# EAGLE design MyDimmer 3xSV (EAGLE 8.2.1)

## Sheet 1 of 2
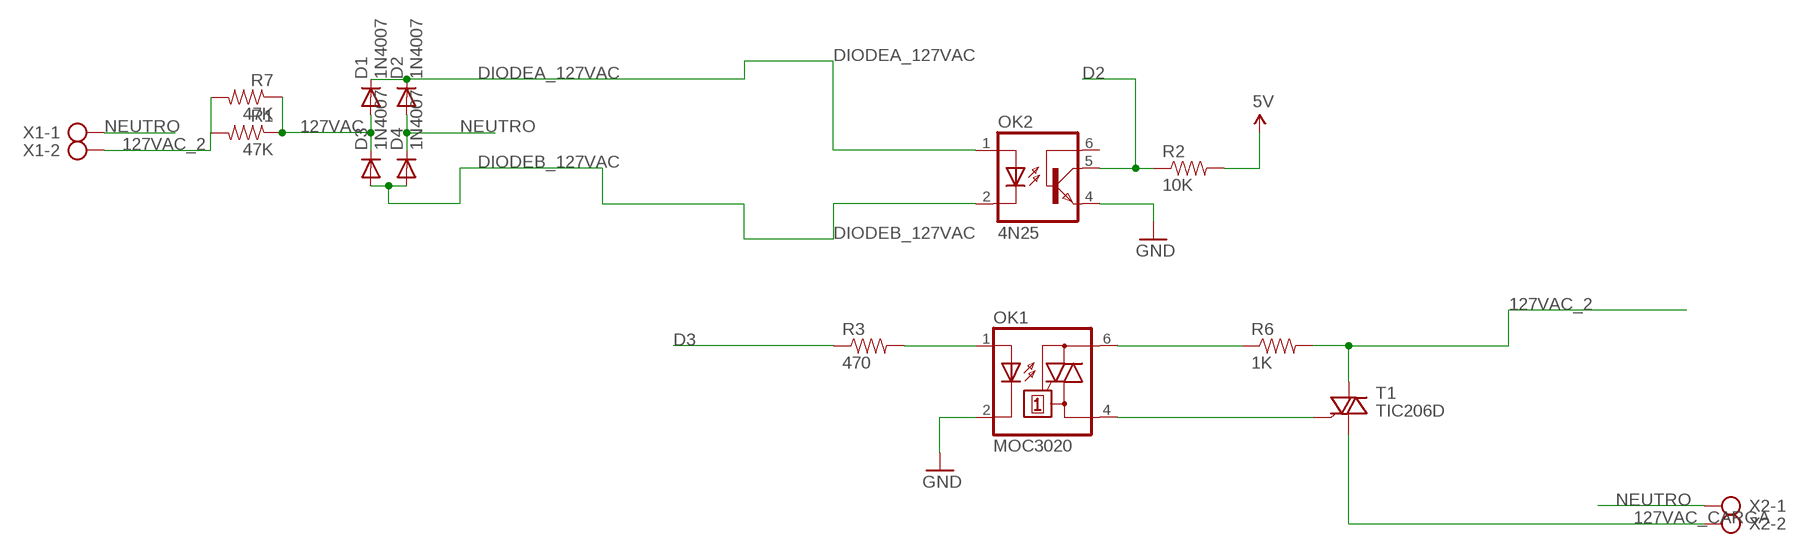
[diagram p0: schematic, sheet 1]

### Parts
D1  1N4007  1N4004  [DO41-10]
D2  1N4007  1N4004  [DO41-10]
D3  1N4007  1N4004  [DO41-10]
D4  1N4007  1N4004  [DO41-10]
OK1  MOC3020  MOC3021M  [DIL06]
OK2  4N25  4N25M  [DIL06]
R1  47K  RESISTORPTH-1/4W  [AXIAL-0.4]
R2  10K  RESISTORPTH-1/4W  [AXIAL-0.4]
R3  470  RESISTORPTH-1/4W  [AXIAL-0.4]
R6  1K  RESISTORPTH-1/4W  [AXIAL-0.4]
R7  47K  RESISTORPTH-1/4W  [AXIAL-0.4]
T1  TIC206D  TIC206M  [TO220BV]
X1  AK500/2-H  [AK500/2-H]
X2  AK500/2-H  [AK500/2-H]

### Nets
5V: R2.P$2 ; also sheet 2
127VAC: D1.A D3.C R1.P$1 R7.P$1
127VAC_2: R1.P$2 R6.P$2 R7.P$2 T1.T2(A2) X1.2
127VAC_CARGA: T1.T1(A1) X2.2
D2: OK2.5(COL) R2.P$1 ; also sheet 2
D3: R3.P$1 ; also sheet 2
DIODEA_127VAC: D1.C D2.C OK2.1(A)
DIODEB_127VAC: D3.A D4.A OK2.2(C)
GND: OK1.2(C) OK2.4(EMI) ; also sheet 2
N$2: OK1.6(A2) R6.P$1
N$5: OK1.4(A1) T1.G
N$7: OK1.1(A) R3.P$2
NEUTRO: D2.A D4.C X1.1 X2.1
Unconnected: OK2.6(BAS)

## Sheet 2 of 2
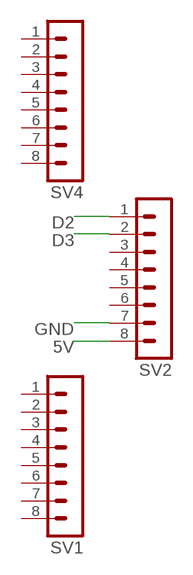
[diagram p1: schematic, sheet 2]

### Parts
SV1  MA08-1  [MA08-1]
SV2  MA08-1  [MA08-1]
SV4  MA08-1  [MA08-1]

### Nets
5V: SV2.8 ; also sheet 1
D2: SV2.1 ; also sheet 1
D3: SV2.2 ; also sheet 1
GND: SV2.7 ; also sheet 1
Unconnected: SV1.1 SV1.2 SV1.3 SV1.4 SV1.5 SV1.6 SV1.7 SV1.8 SV2.3 SV2.4 SV2.5 SV2.6 SV4.1 SV4.2 SV4.3 SV4.4 SV4.5 SV4.6 SV4.7 SV4.8

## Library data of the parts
D1-D4 = adafruit:1N4004: DIODE
OK1 = optocoupler:MOC30*M: RANDOM-PHASE OPTOISOLATORS TRIAC DRIVER OUTPUT Source: http://www.fairchildsemi.com MOC3020-M.pdf; MF: FAIRCHILD SEMICONDUCTOR; MPN: MOC3021-M; OC_FARNELL: 1021365; OC_NEWARK: 95B7895
OK2 = optocoupler:4N*?M: General Purpose 6-Pin Phototransistor Optocouplers Source: http://www.fairchildsemi.com/ds/4N/4N35-M.pdf; MPN: 4N25-M; OC_FARNELL: 1021349; OC_NEWARK: 98K9084
R1-R3 R6 R7 = SparkFun-Resistors:RESISTOR: Resistor
SV1 SV2 SV4 = con-lstb:MA08-1: PIN HEADER
T1 = triac:TIC206: TRIAC Source: http://www.bourns.com/pdfs/tic206.pdf
X1 X2 = con-ptr500:AK500/2-H: CONNECTOR; OC_FARNELL: unknown; OC_NEWARK: unknown

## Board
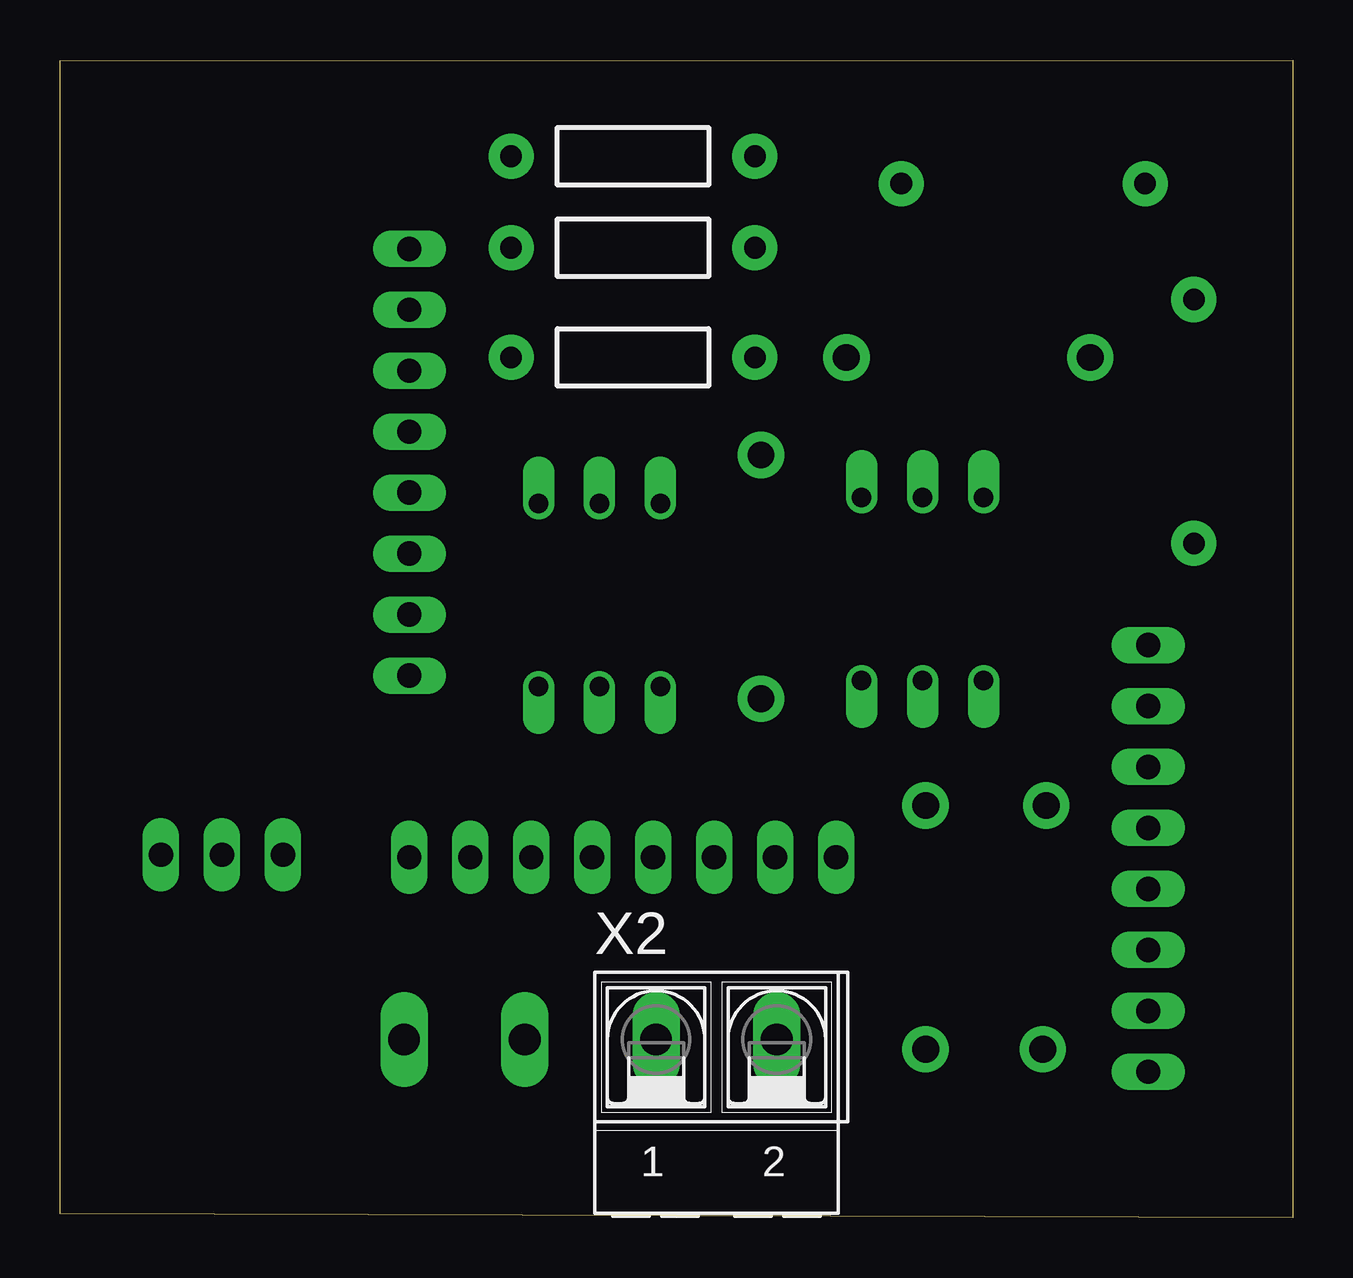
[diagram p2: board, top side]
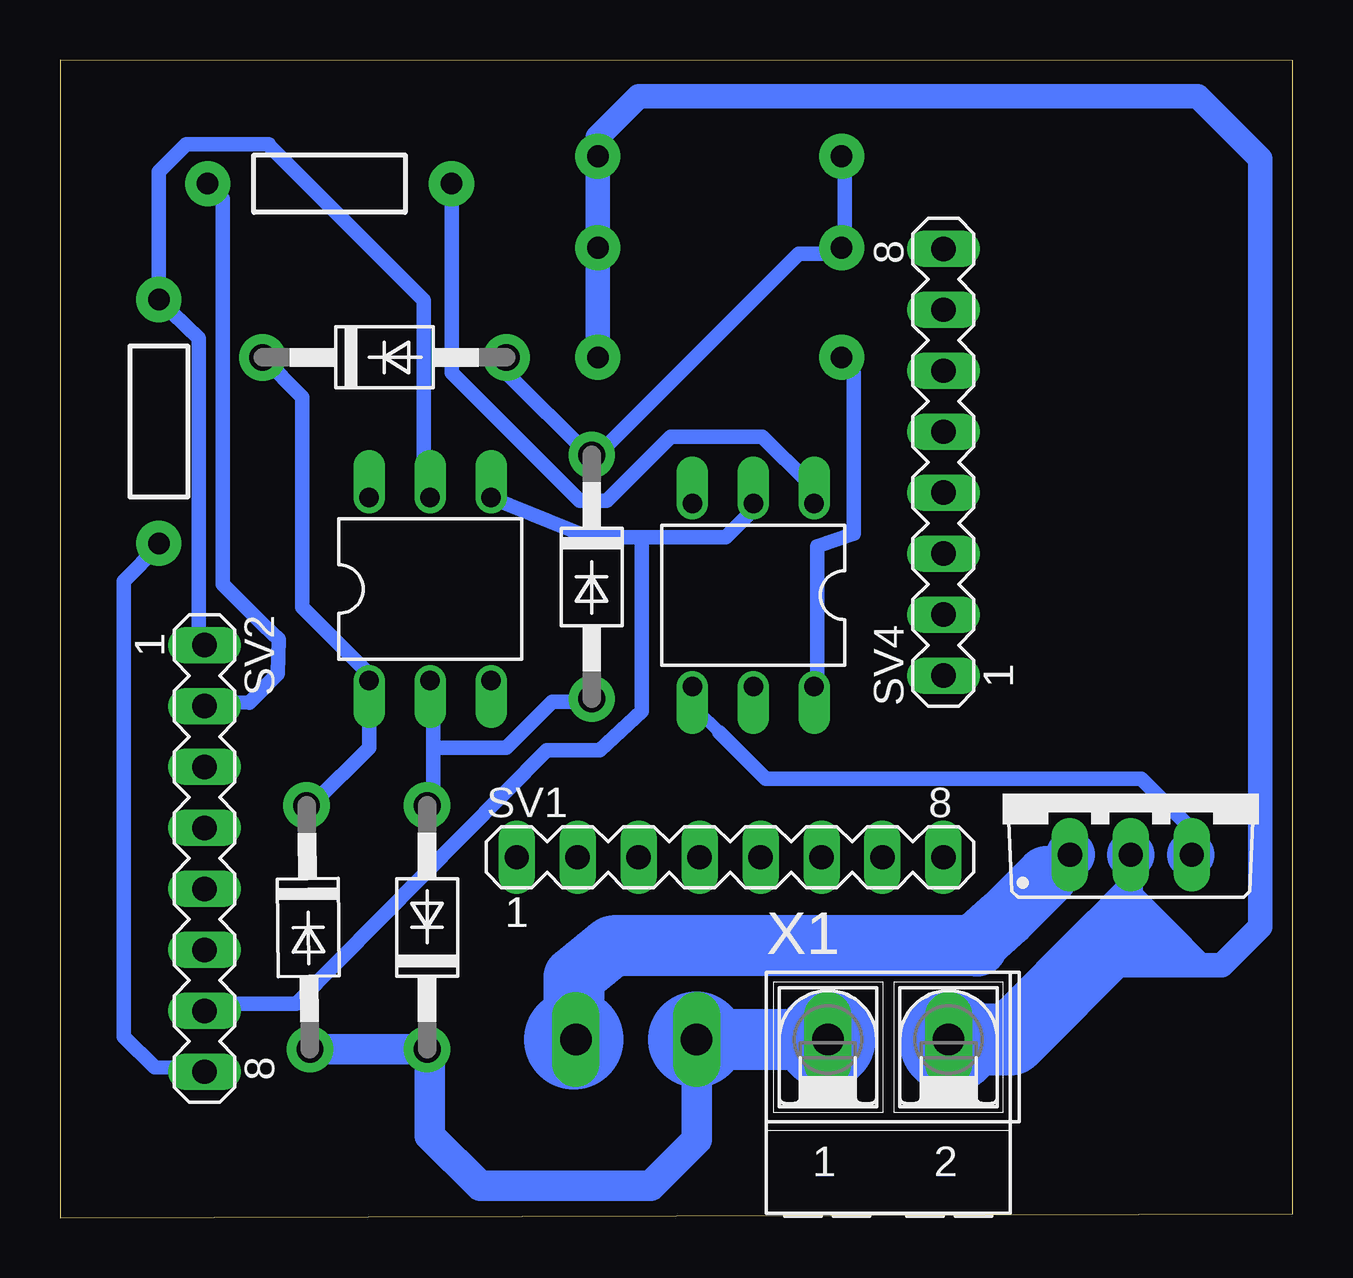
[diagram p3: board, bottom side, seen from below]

Size 51.36 x 48.25 mm. Coordinates in mm from the lower left corner, seen from the top.
Outline: 51.36,0 0,0.17 0,48.22 51.36,48.25 51.36,0
Copper layers (1*16): Top 0.035mm / dielectric 1.5mm / Bottom 0.035mm
Design rules "default": minimum track width 10mil, minimum drill 24mil, track to track 20mil, track to pad 20mil, pad to pad 20mil, via to via 20mil, smd to smd 8mil, copper to edge 40mil, drill to drill 8mil, minimum pad ring 10mil, minimum via ring 8mil, stop-mask expansion 4mil, vias tented up to drill 0mil, thermal gap 10mil

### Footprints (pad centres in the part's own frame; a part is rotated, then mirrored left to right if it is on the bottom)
DO41-10 = drill 1.118 pad 1.93: A 5.08,0; C -5.08,0
DIL06 = drill 0.813 offset: 1 -2.54,-3.81; 2 0,-3.81; 3 2.54,-3.81; 4 2.54,3.81; 5 0,3.81; 6 -2.54,3.81
AXIAL-0.4 = drill 0.9 pad 1.88: P$1 -5.08,0; P$2 5.08,0
MA08-1 = drill 1.016 long: 1 -8.89,0; 2 -6.35,0; 3 -3.81,0; 4 -1.27,0; 5 1.27,0; 6 3.81,0; 7 6.35,0; 8 8.89,0
TO220BV = drill 1.016 long: G 2.54,-2.54; T1 -2.54,-2.54; T2 0,-2.54
AK500/2-H = drill 1.321 long: 1 -2.515,0; 2 2.515,0

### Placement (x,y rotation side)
D1  37.85,35.85 0 bottom
D2  41.02,12.11 270.8 bottom
D3  29.21,26.71 270 bottom
D4  36.07,12.11 90 bottom
OK1  22.48,25.95 180 bottom
OK2  35.94,26.2 0 bottom
R1  23.88,44.24 0 top
R2  47.24,33.19 270 bottom
R3  40.13,43.09 0 bottom
R6  23.88,35.85 0 top
R7  23.88,40.43 0 top
SV1  23.44,15.03 0 bottom
SV2  45.34,14.98 270 bottom
SV4  14.55,31.49 90 bottom
T1  6.75,17.67 0 bottom
X1  16.85,7.43 0 bottom
X2  27.35,7.43 0 top

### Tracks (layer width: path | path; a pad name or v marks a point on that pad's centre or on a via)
5V
  Bottom 0.254: 47.24,27.98 R2.P$2
  Bottom 0.61: 47.24,27.98 47.62,27.6 | SV2.8 45.72,6.26 47.42,6.27 48.71,7.56 48.71,26.54 47.24,28 R2.P$2
127VAC
  Bottom 0.254: 29.34,31.79 D3.C 28.95,31.79 | 19.05,40.17 R7.P$1
  Bottom 0.61: R7.P$1 18.67,40.55 18.67,43.98 R1.P$1 | 29.34,31.79 32.77,35.22 D1.A | 19.05,40.17 20.57,40.17 28.95,31.79
127VAC_2
  Bottom 0.508: T1.T2 | 6.75,12.04 6.85,12.04
  Bottom 1.016: 5.25,10.54 7.65,10.54 | 4.65,10.54 2.95,10.54 1.35,12.13 1.35,44.13 3.95,46.73 27.25,46.73 28.95,45.03 R1.P$2 | 4.65,10.54 5.25,10.54 | 5.25,10.54 6.75,12.04 T1.T2 | 8.35,10.54 6.85,12.04 | 4.65,10.54 4.65,11.33 6.65,13.33 | T1.T2 6.75,12.44 11.75,7.43 | R1.P$2 R6.P$2 | R1.P$2 28.95,44.03 29.05,43.93 | R7.P$2 R1.P$2
  Bottom 3: X1.2 11.75,7.43 7.45,11.73
127VAC_CARGA
  Bottom 0.61: T1.T1 9.29,15 | 29.95,7.52 X2.2
  Bottom 0.813: 9.29,15 13.15,11.33
  Bottom 2.54: 13.15,11.33 28.35,11.33 29.95,10.04 29.95,7.52
D2
  Bottom 0.254: 45.59,24.17 SV2.1
  Bottom 0.61: 36.19,30.27 OK2.5 36.21,30.28 36.21,38.23 42.67,44.7 42.67,44.74 46.1,44.74 47.24,43.6 R2.P$1 45.59,36.66 45.59,24.17
D3
  Bottom 0.61: R3.P$1 44.58,42.46 44.58,26.4 42.85,24.68 42.25,24.11 42.3,22.67 43.48,21.47 45.34,21.5 SV2.2
DIODEA_127VAC
  Bottom 0.254: 40.77,17.31 D2.C | 38.48,22.65 OK2.1
  Bottom 0.61: OK2.1 38.48,19.6 40.77,17.31 | 38.48,22.65 41.27,25.44 41.27,34.2 D1.C
DIODEB_127VAC
  Bottom 0.254: 35.81,22.27 OK2.2 | 29.34,21.5 D3.A
  Bottom 0.61: 35.81,19.6 35.81,17.31 D4.A | 35.81,19.6 35.81,22.27 | 29.34,21.5 30.86,21.5 32.77,19.6 35.81,19.6
GND
  Bottom 0.254: 22.48,29.51 OK1.2 | 45.34,8.93 SV2.7
  Bottom 0.61: 33.15,29.89 OK2.4 29.34,28.36 27.13,28.36 | 27.13,28.36 23.62,28.36 22.48,29.51 | 45.34,8.93 41.53,8.93 31.08,19.48 28.87,19.48 27.13,21.12 27.13,28.36
N$1
  Bottom 1.016: 8.15,12.23 8.15,12.44 6.85,13.73
N$2
  Bottom 0.254: 19.81,22.27 OK1.6
  Bottom 0.61: 19.81,22.27 19.81,27.98 18.29,28.51 18.29,35.22 18.67,35.6 R6.P$1
N$3
  Bottom 2.54: 12.95,11.63 11.95,12.54 10.25,14.23
N$4
  Bottom 1.016: 5.35,11.83 5.15,11.83 3.95,10.63
N$5
  Bottom 0.508: 24.76,21.12 23.9,20.26 23.9,20.23 | 4.25,15.18 T1.G
  Bottom 0.61: 24.76,21.12 24.76,21.89 OK1.4 | 23.9,20.23 21.97,18.3 6.31,18.3 4.25,16.24 4.25,15.18
N$7
  Bottom 0.61: R3.P$2 35.05,35.22 29.72,29.89 28.57,29.89 25.91,32.55 22.1,32.55 20.19,30.65 20.19,29.89 OK1.1
NEUTRO
  Bottom 0.61: D4.C 35.66,7.43 | D2.A
  Bottom 1.016: 35.95,6.91 D4.C
  Bottom 1.27: D4.C D2.A | 35.95,6.91 35.95,3.43 33.85,1.33 26.75,1.33 24.84,3.25 X2.1
  Bottom 2.54: X1.1 X2.1
(copper drawn outside any net)
  shapes: Bottom circle x7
